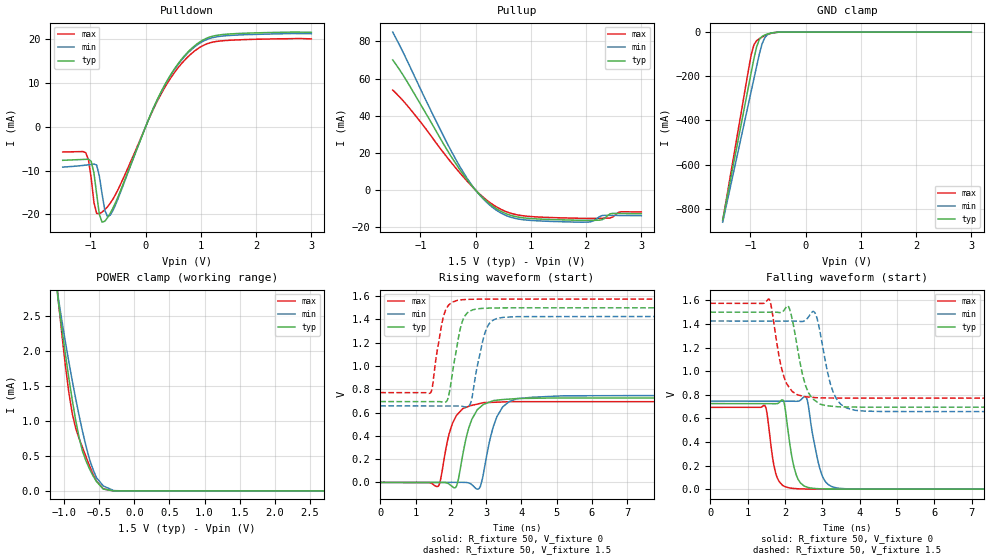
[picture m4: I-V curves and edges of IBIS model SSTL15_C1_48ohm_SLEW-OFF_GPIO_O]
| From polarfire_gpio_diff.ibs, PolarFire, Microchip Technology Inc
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|   Model SSTL15_C1_48ohm_SLEW-OFF_GPIO_O
[Model]   SSTL15_C1_48ohm_SLEW-OFF_GPIO_O
Model_type   Output
Polarity   Non-Inverting
Enable   Active-High
Vmeas =   0.75
Cref =   5p
Rref =   50
Vref =   0.75
|   typ   min   max
C_comp_pullup   2.605e-12   2.605e-12   2.76e-12
C_comp_pulldown  2.605e-12   2.605e-12   2.76e-12
[Temperature Range]  25C   100C   -40C
[Voltage Range]  1.5   1.425   1.575
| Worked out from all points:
|   slope of the pulldown table from 0 to 0.225 V, typ, clamps not added: 34.2 ohm
|   slope of the pullup table from 0 to 0.225 V, typ, clamps not added: 34 ohm
|   GND clamp passes 1 mA (typ) near -0.52 V on its own axis
|   POWER clamp passes 1 mA (typ) near -0.84 V on its own axis
|   rising waveform, R_fixture 50, V_fixture 0: 20-80 % time 383ps typ, 401ps min, 350ps max; typ from 0 V to 0.725 V
|   rising waveform, R_fixture 50, V_fixture 1.5: 20-80 % time 280ps typ, 308ps min, 259ps max; typ from 0.694 V to 1.5 V
|   falling waveform, R_fixture 50, V_fixture 0: 20-80 % time 233ps typ, 283ps min, 193ps max; typ from 0.725 V to 0 V
|   falling waveform, R_fixture 50, V_fixture 1.5: 20-80 % time 324ps typ, 330ps min, 295ps max; typ from 1.5 V to 0.694 V
[GND Clamp]
| Voltage   I(typ)   I(min)   I(max)
-1.5V     -849.7mA   -860.2mA   -853.5mA
-1.034V   -246.6mA   -324.3mA   -170.7mA
-984.4mV  -183.1mA   -267.7mA   -102.9mA
-935.2mV  -119.9mA   -211.2mA   -57.59mA
-885.9mV  -66.33mA   -154.7mA   -38.94mA
-836.7mV  -33.59mA   -99.09mA   -29.82mA
-787.5mV  -19.44mA   -53.53mA   -22.49mA
-738.3mV  -12.87mA   -24.95mA   -16.13mA
-689.1mV  -8.545mA   -11.57mA   -10.81mA
-590.6mV  -2.947mA   -3.067mA   -3.621mA
-393.7mV  -37.64uA   -63.17uA   -40.12uA
3V        0A         0A         0A
[POWER Clamp]
| Voltage   I(typ)   I(min)   I(max)
-1.5V     10.9mA     9.757mA    12.4mA
-1.181V   3.55mA     3.502mA    3.75mA
-1.083V   2.694mA    2.748mA    2.703mA
-984.4mV  1.956mA    2.133mA    1.792mA
-935.2mV  1.615mA    1.848mA    1.408mA
-836.7mV  1.007mA    1.316mA    894.8uA
-738.3mV  562.1uA    843.7uA    616.9uA
-639.8mV  314.2uA    451.1uA    357.6uA
-541.4mV  134.7uA    190.1uA    142.2uA
-443mV    26.83uA    70.8uA     28.29uA
-147.7mV  138.9nA    173.8nA    970.8pA
3V        0A         0A         0A
[Pullup]
| Voltage   I(typ)   I(min)   I(max)
-1.5V     70.01mA    84.98mA    53.82mA
-1.181V   55.46mA    66mA       43.49mA
-295.3mV  11.42mA    13.18mA    9.637mA
0V        -138.7nA   12.43uA    20.68uA
328.1mV   -8.987mA   -9.76mA    -8.073mA
656.2mV   -13.72mA   -14.73mA   -12.6mA
1.125V    -15.5mA    -16.5mA    -14.43mA
2.041V    -16.26mA   -17.17mA   -15.22mA
2.288V    -15.94mA   -13.69mA   -15.12mA
2.386V    -13.79mA   -13.55mA   -15.06mA
2.632V    -12.56mA   -13.64mA   -11.62mA
3V        -12.67mA   -13.76mA   -11.72mA
[Pulldown]
| Voltage   I(typ)   I(min)   I(max)
-1.5V     -7.654mA   -9.205mA   -5.749mA
-1.083V   -7.43mA    -8.749mA   -5.909mA
-984.4mV  -7.883mA   -8.59mA    -11.7mA
-935.2mV  -10.5mA    -8.502mA   -17.22mA
-885.9mV  -15.31mA   -8.737mA   -19.78mA
-836.7mV  -20.02mA   -11.27mA   -19.87mA
-738.3mV  -21.59mA   -19.05mA   -18.94mA
-590.6mV  -18.57mA   -19.11mA   -16.51mA
281.2mV   8.019mA    7.924mA    7.527mA
843.8mV   18.05mA    17.82mA    16.9mA
1.359V    21.05mA    20.71mA    19.64mA
3V        21.6mA     21.29mA    20.11mA
[Ramp]
dV/dt_r   0.435212/0.383072n  0.447544/0.40119n  0.416049/0.349615n
dV/dt_f   0.483314/0.323801n  0.460744/0.330442n  0.482132/0.295487n
R_load = 50
[Rising Waveform]
R_fixture = 50
V_fixture = 0
V_fixture_min = 0
V_fixture_max = 0
| Time   V(typ)   V(min)   V(max)
0s        14.78nV    20.59nV    20.51nV
1.636ns   -677.1uV   642.8uV    -34.32mV
1.957ns   -15.22mV   768.9uV    421.9mV
2.13ns    -45.11mV   836.8uV    556.9mV
2.512ns   469.6mV    -4.66mV    654.5mV
2.774ns   630.2mV    -57.95mV   674.4mV
2.925ns   670.2mV    74.06mV    685.2mV
3.309ns   706.4mV    564.9mV    689.3mV
3.879ns   720.3mV    718.8mV    693.7mV
10ns      725.4mV    745.9mV    693.4mV
[Rising Waveform]
R_fixture = 50
V_fixture = 1.5
V_fixture_min = 1.425
V_fixture_max = 1.575
| Time   V(typ)   V(min)   V(max)
0s        694.5mV    657.1mV    771.4mV
1.426ns   693.9mV    656.6mV    770mV
1.752ns   691mV      656.4mV    1.372V
1.906ns   709.2mV    656.4mV    1.509V
2.197ns   1.206V     656.3mV    1.565V
2.352ns   1.402V     652mV      1.57V
2.549ns   1.472V     671.2mV    1.573V
2.969ns   1.496V     1.285V     1.575V
3.306ns   1.499V     1.408V     1.575V
10ns      1.5V       1.425V     1.575V
[Falling Waveform]
R_fixture = 50
V_fixture = 0
V_fixture_min = 0
V_fixture_max = 0
| Time   V(typ)   V(min)   V(max)
0s        725.3mV    745.9mV    693.4mV
1.463ns   724.6mV    745.4mV    706.4mV
1.752ns   724.5mV    745.3mV    134.2mV
1.966ns   743.7mV    745.3mV    27.31mV
2.105ns   440mV      745.2mV    11.43mV
2.306ns   116.9mV    744.8mV    4.263mV
2.581ns   18.32mV    768.8mV    1.259mV
2.97ns    2.642mV    137mV      277.6uV
3.354ns   463uV      12.47mV    -1.484uV
10ns      645nV      3.921uV    819.8nV
[Falling Waveform]
R_fixture = 50
V_fixture = 1.5
V_fixture_min = 1.425
V_fixture_max = 1.575
| Time   V(typ)   V(min)   V(max)
0s        1.5V       1.425V     1.575V
1.573ns   1.499V     1.424V     1.611V
1.895ns   1.498V     1.424V     1.041V
2.07ns    1.554V     1.424V     882mV
2.176ns   1.465V     1.424V     835mV
2.528ns   904.1mV    1.427V     783.1mV
2.809ns   749.7mV    1.491V     775.9mV
3.211ns   704.2mV    897.3mV    772.5mV
3.661ns   696.7mV    686.1mV    771.5mV
10ns      694.5mV    657.1mV    771.4mV
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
